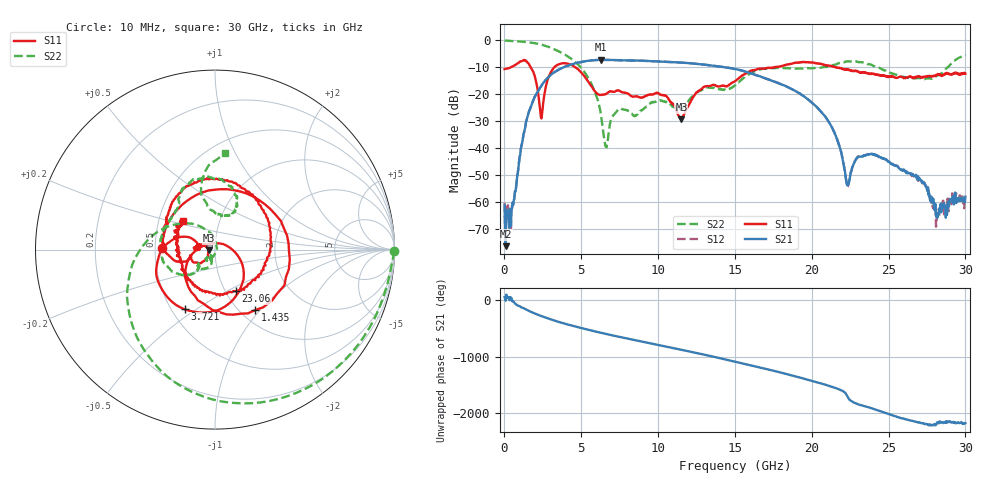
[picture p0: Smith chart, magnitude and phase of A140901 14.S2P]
!  2-Port S-parameters saved by WinCal
! VAR MeasName=S-Parameters (CALIBRATED_DATA) read from VNA (N5244A)
! VAR MeasDate=11/3/2014 9:27:50 AM
! VAR NAME=A140901 14
! VAR FILENAME=A140901 14.S2P
! VAR DATE=11/3/2014 9:27:50 AM
! VAR PHYS_PORTS=1,2
# Hz S RI R 50
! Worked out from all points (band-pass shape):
!   801 points, 10 MHz to 30 GHz, reference 50 ohm
!   highest |S21| = -7.21 dB at 6.27 GHz (marker M1); lowest = -76.4 dB at 84.97 MHz (marker M2)
!   |S21| within 3 dB of the highest: 3.759 GHz to 14.62 GHz (10.86 GHz wide, 118 % of centre)
!   lowest |S11| = -29.3 dB at 11.52 GHz (marker M3), VSWR 1.07, Z = 46.7 - j0.298 ohm
!   |S11| at or under -10 dB: 1.708 GHz to 3.243 GHz (1.535 GHz wide, 62 % of centre); 4.61 GHz to 17.56 GHz (12.95 GHz wide, 117 % of centre); 21.64 GHz to end of sweep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
!   |S22| runs from -39.7 to 0.0 dB; largest |S21 - S12| = 0.0022
!   S11 on the Smith chart (normalised r, x): 10 MHz: 0.55, +0.01; 1.435 GHz: 1.17, -0.94; 3.721 GHz: 0.58, -0.45; 23.06 GHz: 1.12, -0.56; 30 GHz: 0.67, +0.23
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1e7  -0.2929 0.00893  0.000449 0.000736  -2.41e-06 -0.000969  0.9968 -0.00832
8.4975e7  -0.2893 0.066  0.00015 -2.06e-05  2.57e-05 0.000265  0.988 -0.0623
4.5985e8  -0.1034 0.3048  0.000571 0.000463  0.000789 0.000417  0.9298 -0.2872
1.434525e9  0.2249 -0.3363  -0.0318 -0.00734  -0.0318 -0.00723  0.5601 -0.7445
2.4092e9  0.0065 0.035  0.0253 0.1431  0.025 0.1428  -0.0226 -0.8324
3.721262e9  -0.1687 -0.3327  0.2392 -0.1895  0.239 -0.1889  -0.4811 -0.3352
5.033325e9  -0.2407 0.0518  -0.2778 -0.2875  -0.2778 -0.2873  -0.2727 0.1233
6.270412e9  -0.0966 0.0116  -0.3532 0.2556  -0.3535 0.2551  0.00303 0.0425
6.6078e9  -0.1007 0.000441  -0.238 0.3634  -0.2378 0.363  0.0107 -0.000968
7.35755e9  -0.1175 0.0105  0.0852 0.4214  0.0846 0.421  -0.0269 -0.0426
8.482175e9  -0.0896 0.0169  0.4096 0.1061  0.4092 0.1067  -0.0232 -0.0321
1.001916e10  -0.1041 0.0128  0.1243 -0.3872  0.1237 -0.3868  -0.0456 -0.0629
1.151866e10  -0.0343 -0.00319  -0.3561 -0.1503  -0.3552 -0.15  -0.0239 -0.0484
1.328058e10  -0.1272 -0.0615  -0.0581 0.3422  -0.0579 0.3405  -0.0824 -0.1046
1.5005e10  -0.1619 -0.0649  0.2927 -0.0316  0.2923 -0.0324  -0.0947 -0.1114
2.002832e10  0.0943 0.3789  0.0675 0.014  0.0677 0.0143  -0.2241 0.2018
2.145285e10  0.3103 0.0916  -0.0054 -0.0193  -0.00505 -0.0195  -0.203 0.2869
2.231506e10  0.2572 -0.1332  -0.000441 0.00199  -0.000351 0.00189  -0.1236 0.387
2.306481e10  0.1177 -0.2317  0.00452 -0.00515  0.00466 -0.00518  0.00182 0.3972
2.501416e10  -0.1675 -0.1228  -0.00447 0.00343  -0.00431 0.00351  0.1174 0.2333
2.812562e10  -0.2176 0.0649  0.000427 -0.000303  0.000409 -0.000184  -0.0175 0.2176
3e10  -0.1792 0.1605  0.0012 -0.000352  0.000835 -0.000549  0.0559 0.5379
